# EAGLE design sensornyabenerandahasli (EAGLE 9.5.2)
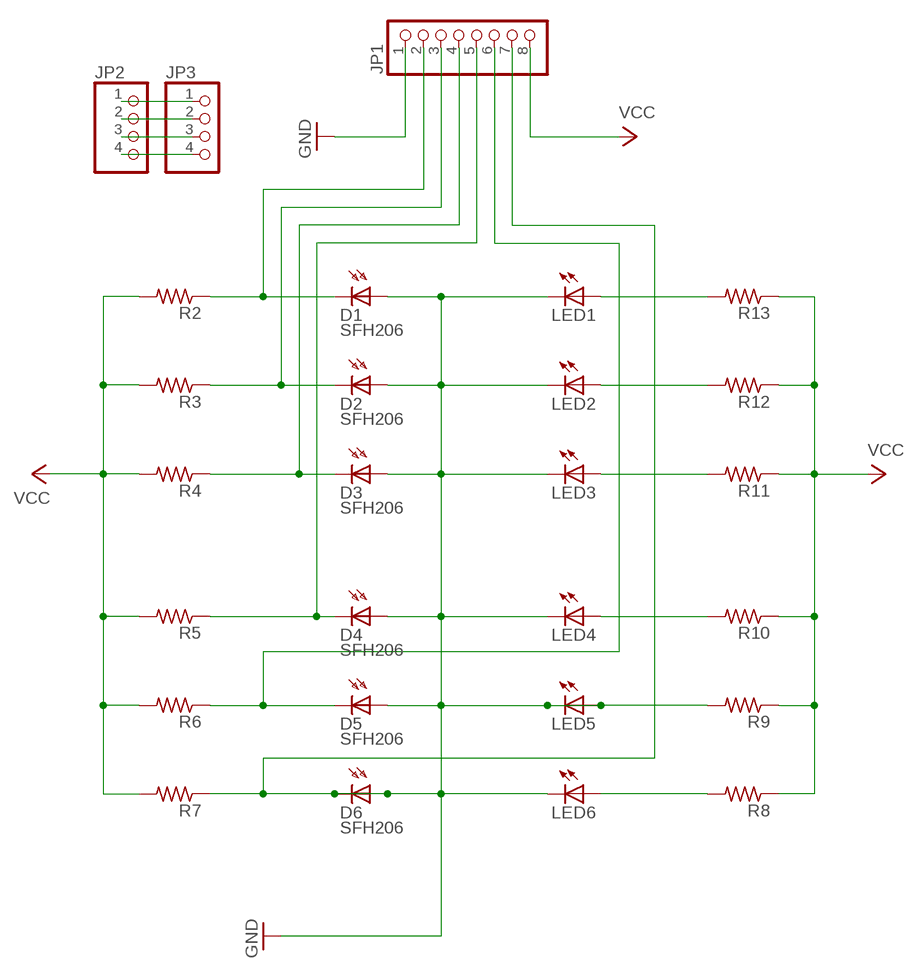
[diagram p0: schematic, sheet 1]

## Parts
D1  SFH206  [SFH206]
D2  SFH206  [SFH206]
D3  SFH206  [SFH206]
D4  SFH206  [SFH206]
D5  SFH206  [SFH206]
D6  SFH206  [SFH206]
JP1  PINHD-1X8  [1X08]
JP2  PINHD-1X4  [1X04]
JP3  PINHD-1X4  [1X04]
LED1  LED5MM  [LED5MM]
LED2  LED5MM  [LED5MM]
LED3  LED5MM  [LED5MM]
LED4  LED5MM  [LED5MM]
LED5  LED5MM  [LED5MM]
LED6  LED5MM  [LED5MM]
R2  R-US_0204/7  [0204/7]
R3  R-US_0204/7  [0204/7]
R4  R-US_0204/7  [0204/7]
R5  R-US_0204/7  [0204/7]
R6  R-US_0204/7  [0204/7]
R7  R-US_0204/7  [0204/7]
R8  R-US_0204/7  [0204/7]
R9  R-US_0204/7  [0204/7]
R10  R-US_0204/7  [0204/7]
R11  R-US_0204/7  [0204/7]
R12  R-US_0204/7  [0204/7]
R13  R-US_0204/7  [0204/7]

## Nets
GND: D1.A D2.A D3.A D4.A D5.A D6.A D6.K(C) JP1.1 JP1.7 LED1.K(C) LED2.K(C) LED3.K(C) LED4.K(C) LED5.A LED5.K(C) LED6.K(C) R7.1 R9.2
N$1: D1.K(C) JP1.2 R2.1
N$2: JP2.1 JP3.1
N$3: LED1.A R13.2
N$4: D5.K(C) JP1.6 R6.1
N$5: JP2.2 JP3.2
N$6: D2.K(C) JP1.3 R3.1
N$7: JP2.3 JP3.3
N$8: LED2.A R12.2
N$9: D3.K(C) JP1.4 R4.1
N$10: JP2.4 JP3.4
N$11: LED3.A R11.2
N$12: D4.K(C) JP1.5 R5.1
N$14: LED4.A R10.2
N$15: LED6.A R8.2
VCC: JP1.8 R2.2 R3.2 R4.2 R5.2 R6.2 R7.2 R8.1 R9.1 R10.1 R11.1 R12.1 R13.1

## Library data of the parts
D1-D6 = opto-trans-siemens:SFH206: PHOTO DIODE; MPN: SFH206K; OC_FARNELL: 1212741; OC_NEWARK: 01M8807
JP1 = pinhead:PINHD-1X8: PIN HEADER
JP2 JP3 = pinhead:PINHD-1X4: PIN HEADER
LED1-LED6 = led:LED: LED
R2-R13 = rcl:R-US_: RESISTOR, American symbol; SPICEPREFIX: R

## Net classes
0 default: width 0.635 mm

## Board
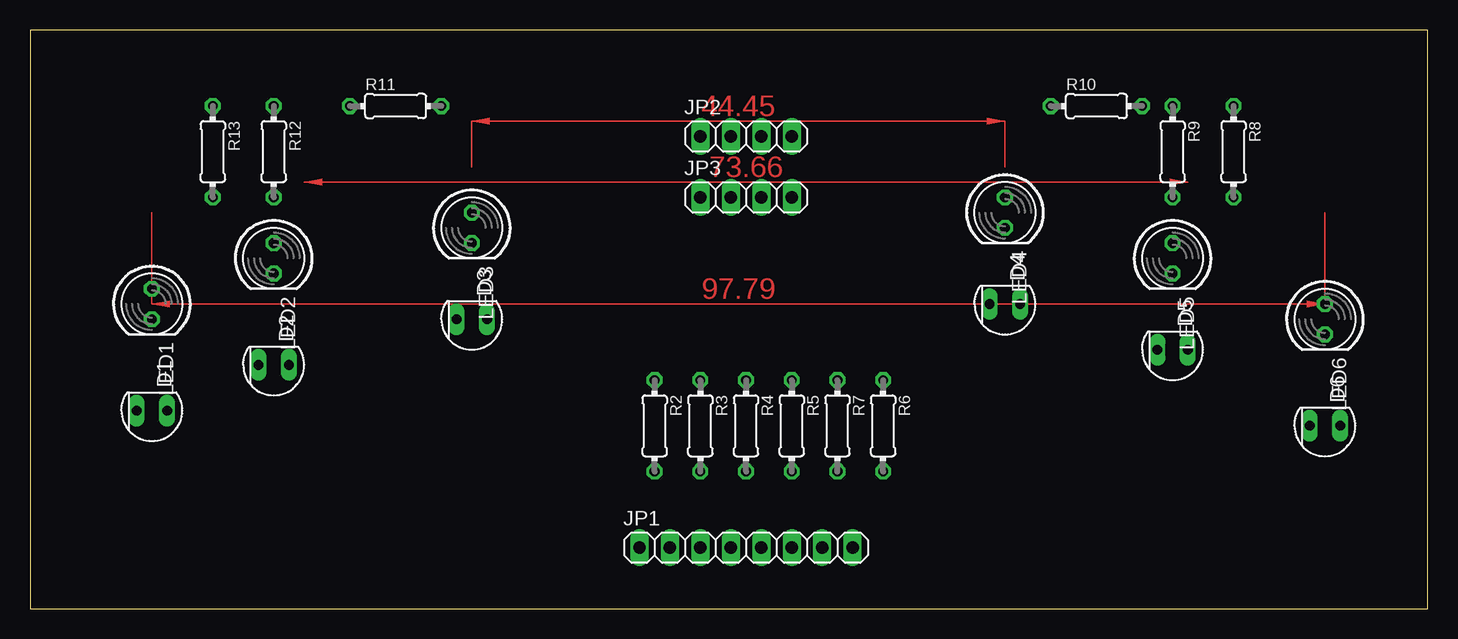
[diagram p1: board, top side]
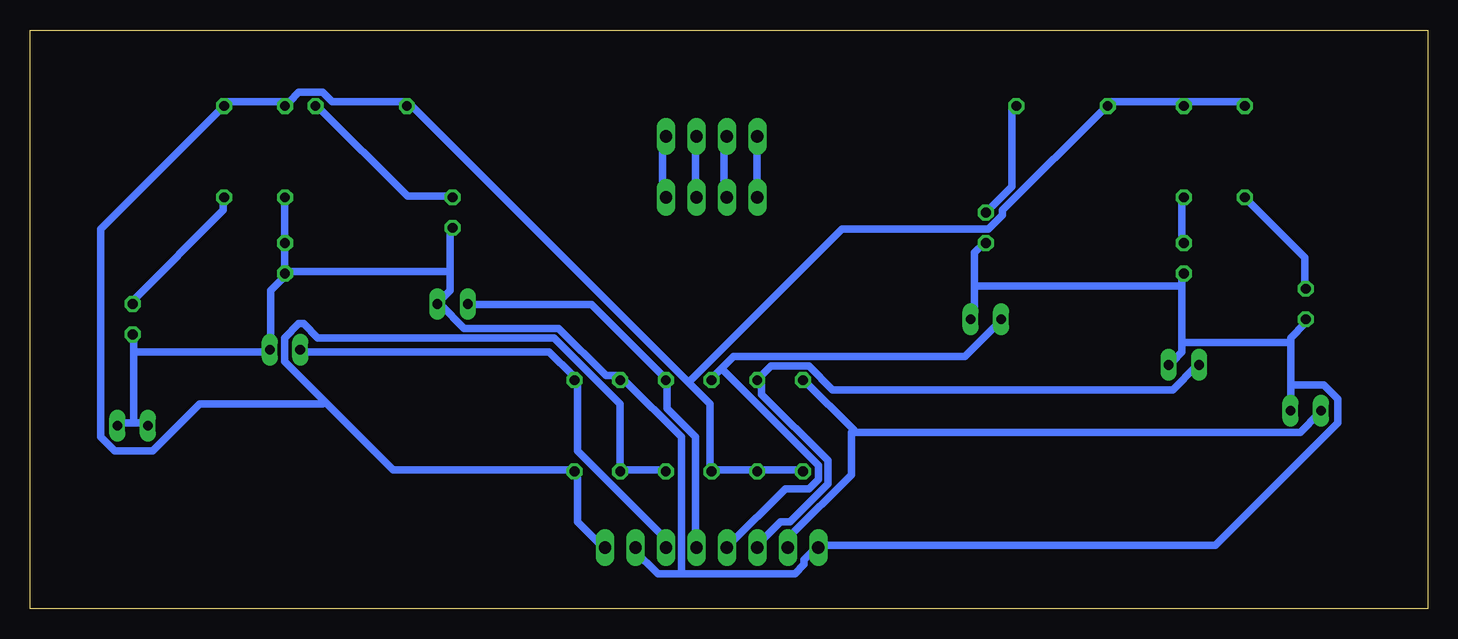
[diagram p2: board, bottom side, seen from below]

Size 116.51 x 48.25 mm. Coordinates in mm from the lower left corner, seen from the top.
Outline: 0,0 116.51,0 116.51,48.25 0,48.25 0,0
Copper layers (1*16): Top 0.035mm / dielectric 1.5mm / Bottom 0.035mm
Design rules "default": minimum track width 6mil, minimum drill 0.35mm, track to track 6mil, track to pad 6mil, pad to pad 6mil, via to via 6mil, smd to smd 6mil, copper to edge 40mil, drill to drill 6mil, minimum pad ring 10mil, minimum via ring 8mil, stop-mask expansion 4mil, vias tented up to drill 0mil, thermal gap 10mil

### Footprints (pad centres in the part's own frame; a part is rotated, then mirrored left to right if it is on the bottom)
SFH206 = drill 0.813 long: A 0,-1.27; K 0,1.27
1X08 = drill 1.016 long: 1 -8.89,0; 2 -6.35,0; 3 -3.81,0; 4 -1.27,0; 5 1.27,0; 6 3.81,0; 7 6.35,0; 8 8.89,0
1X04 = drill 1.016 long: 1 -3.81,0; 2 -1.27,0; 3 1.27,0; 4 3.81,0
LED5MM = drill 0.813 octagon: A -1.27,0; K 1.27,0
0204/7 = drill 0.813 octagon: 1 -3.81,0; 2 3.81,0

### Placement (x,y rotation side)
D1  10.16,16.51 90 top
D2  20.32,20.32 90 top
D3  36.83,24.13 90 top
D4  81.28,25.4 90 top
D5  95.25,21.59 90 top
D6  107.95,15.24 90 top
JP1  59.69,5.08 0 top
JP2  59.69,39.37 0 top
JP3  59.69,34.29 0 top
LED1  10.16,25.4 270 top
LED2  20.32,29.21 270 top
LED3  36.83,31.75 270 top
LED4  81.28,33.02 270 top
LED5  95.25,29.21 270 top
LED6  107.95,24.13 270 top
R2  52.07,15.24 270 top
R3  55.88,15.24 270 top
R4  59.69,15.24 270 top
R5  63.5,15.24 270 top
R6  71.12,15.24 270 top
R7  67.31,15.24 270 top
R8  100.33,38.1 270 top
R9  95.25,38.1 270 top
R10  88.9,41.91 0 top
R11  30.48,41.91 0 top
R12  20.32,38.1 270 top
R13  15.24,38.1 270 top

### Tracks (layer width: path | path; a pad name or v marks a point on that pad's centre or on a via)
GND
  Bottom 0.635: 11.42,22.19 11.42,22.58 10.24,23.76 LED1.K | 11.42,22.19 11.42,18.64 | 11.42,18.64 11.42,16.67 D1.A | 37.8,26.91 37.8,29.67 37.01,30.45 LED3.K | 37.8,26.91 37.8,24.16 D3.A | 20.47,22.19 20.47,21.4 21.26,20.61 D2.A | 20.47,22.19 20.47,26.91 | 20.47,26.91 20.47,27.7 LED2.K | 20.47,26.91 37.8,26.91 | 20.47,22.19 11.42,22.19 | 107.87,15.49 109.06,15.49 D6.A | 107.87,15.49 106.69,15.49 D6.K | 107.87,15.49 107.87,21.4 | 107.87,21.4 107.87,22.58 LED6.K | LED5.K 95.28,28.09 95.28,30.45 LED5.A 95.28,30.85 95.28,34 R9.2 | LED5.K 95.28,27.7 96.46,26.52 96.46,21.79 D5.A 96.85,21.4 107.87,21.4 | 62.2,2.9 64.17,2.9 66.14,4.86 JP1.7 | 62.2,2.9 52.76,2.9 51.97,3.68 51.97,4.08 51.18,4.86 JP1.1 50.79,5.26 17.72,5.26 7.48,15.49 7.48,17.46 8.66,18.64 11.42,18.64 | 81.5,28.09 81.5,26.52 82.28,25.73 D4.A 82.28,25.34 80.31,23.37 72.44,23.37 68.5,19.43 67.32,19.43 R7.1 66.93,19.04 62.2,14.31 62.2,2.9 | 81.5,28.09 81.5,31.64 LED4.K | 81.5,28.09 94.88,28.09 LED5.K
N$1
  Bottom 0.635: 47.84,14.9 51.97,19.04 R2.1 | 47.84,14.9 47.64,14.71 10.63,14.71 9.05,16.28 D1.K | JP1.2 53.15,5.26 53.15,6.05 48.03,11.16 48.03,14.71 47.84,14.9
N$2
  Bottom 0.635: JP3.1 55.91,34.39 55.91,39.12 JP2.1
N$3
  Bottom 0.635: LED1.A 10.24,26.91 10.24,29.27 14.96,34 R13.2
N$4
  Bottom 0.635: JP1.6 63.78,5.26 63.78,6.05 70.87,13.13 70.87,19.04 R6.1 71.26,19.43 73.23,21.4 93.7,21.4 D5.K
N$5
  Bottom 0.635: JP3.2 58.66,34.39 58.66,39.12 JP2.2
N$6
  Bottom 0.635: JP1.3 55.91,5.26 53.94,7.23 53.15,7.23 50,10.38 50,12.34 55.51,17.86 55.51,19.04 R3.1 55.51,19.43 54.72,20.22 51.58,20.22 49.61,18.25 21.26,18.25 19.29,20.22 D2.K
N$7
  Bottom 0.635: JP3.3 61.02,34.39 61.02,39.12 JP2.3
N$8
  Bottom 0.635: LED2.A 20.47,30.85 20.47,34 R12.2
N$9
  Bottom 0.635: 58.86,20.02 59.45,19.43 R4.1 | 58.86,20.02 57.87,21.01 38.58,21.01 35.83,23.76 D3.K | 58.86,20.02 50.79,11.95 50.79,10.77 51.58,9.98 53.54,9.98 58.27,5.26 JP1.4
N$10
  Bottom 0.635: JP3.4 63.78,34.39 63.78,39.12 JP2.4
N$11
  Bottom 0.635: R11.2 34.65,41.87 34.65,35.18 36.61,33.21 LED3.A
N$12
  Bottom 0.635: JP1.5 61.02,5.26 61.02,14.31 63.39,16.67 63.39,19.04 R5.1 63.78,19.43 69.69,25.34 79.92,25.34 D4.K
N$14
  Bottom 0.635: LED4.A 81.5,34.39 85.04,34.39 92.52,41.87 R10.2
N$15
  Bottom 0.635: R8.2 100.39,34 100.39,33.21 107.87,25.73 LED6.A
VCC
  Bottom 0.635: R5.2 63.78,11.56 66.93,11.56 R7.2 67.32,11.56 67.32,17.07 72.83,22.58 92.52,22.58 93.7,23.76 94.09,23.76 95.28,22.58 95.28,20.61 91.93,17.27 | JP1.8 68.9,5.26 70.87,7.23 70.87,11.16 R6.2 71.26,11.56 86.22,11.56 91.93,17.27 | R13.1 15.35,42.27 20.08,42.27 R12.1 20.47,42.27 26.38,42.27 R11.1 26.77,41.87 35.43,33.21 35.43,32.82 36.61,31.64 48.82,31.64 61.61,18.84 | R2.2 52.36,11.56 55.51,11.56 R3.2 55.91,11.56 59.45,11.56 R4.2 59.84,11.56 59.84,17.07 61.61,18.84 | 61.61,18.84 85.04,42.27 R10.1 85.43,42.27 91.34,42.27 92.13,43.05 94.09,43.05 94.88,42.27 R9.1 95.28,42.27 100,42.27 R8.1 100.39,41.87 110.63,31.64 110.63,14.31 109.45,13.13 106.3,13.13 102.36,17.07 92.13,17.07 91.93,17.27
(copper drawn outside any net)
  shapes: Top area x3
